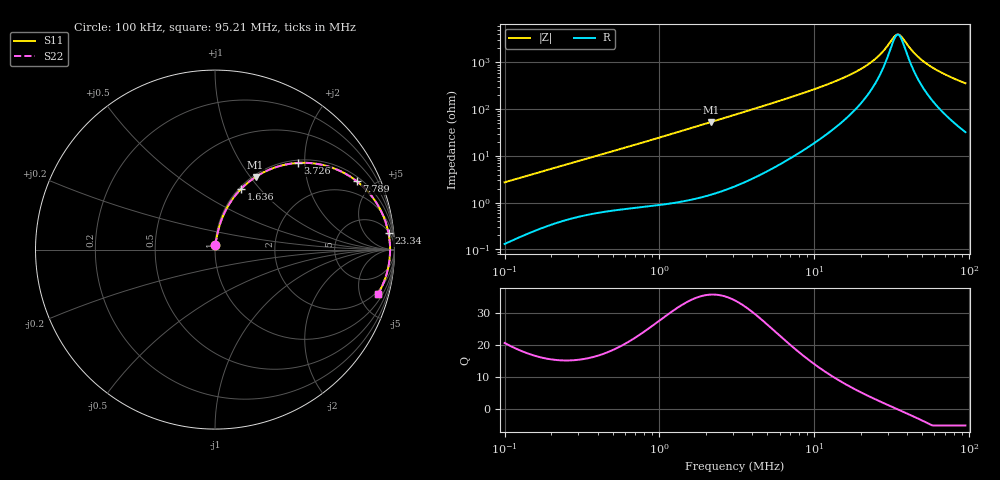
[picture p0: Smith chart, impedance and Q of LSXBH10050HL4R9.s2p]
! LSXBH10050HL4R9  S-PARAMETER MODEL  ( General Type )
! Model Generated by TAIYO YUDEN Corporation (http://www.ty-top.com)
! Version 3.0
! TAIYO YUDEN Control No. 180118NI43SB-FBB
! Copyright(c) 2007 TAIYO YUDEN CO.,LTD. All Rights Reserved.
! Product Description (link to TY-COMPAS)
! https://ds.yuden.co.jp/TYCOMPAS/or/detail?pn=LSXBH10050HL4R9N&u=M
! Products Name : Inductors
! Characteristics :
!  Inductance : 4.9 uH , SRF(min) : 23 MHz , DC Resistance(max) : 0.0195 Ohm
!  Rated Current : Saturation :6600 mA , Temp Rise : 6000 mA (40 degC)
!  Case Size : 10.0 x 9.8 / 0.394 x 0.386 [mm/inch] , Thickness : 5 / 0.197 [mm/inch]
!  (Conditions: Temperature = 25 degC , DC Bias Current/Voltage = 0A / 0V)
! External Node Assignments :
!  1  o---GGG---o  2
! GND o---------o GND
! Frequency Range : 0.1MHz  -  95.211795MHz  [ 402 STEP ]
# MHz S RI R 50
! Freq[MHz].  S11 Real  S11 Imag  S21 Real  S21 Imag  S12 Real  S12 Imag  S22 Real  S22 Imag
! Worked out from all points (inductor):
!   401 points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, 100 kHz to 95.21 MHz, reference 50 ohm
!   read as one part in series: L = 4.29 uH near 103.5 kHz
!   highest Q = 35.9 at 2.153 MHz (marker M1), where L = 3.92 uH
!   self-resonance near 34.84 MHz
!   S11 on the Smith chart (normalised r, x): 100 kHz: 1.00, +0.05; 1.636 MHz: 1.02, +0.81; 3.726 MHz: 1.06, +1.85; 7.789 MHz: 1.22, +4.01; 23.34 MHz: 6, +19; 95.21 MHz: 1.65, -7.16
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0.1  0.00205 0.0271  0.998 -0.0271  0.998 -0.0271  0.00205 0.0271
0.31545  0.0116 0.0796  0.9884 -0.0796  0.9884 -0.0796  0.0116 0.0796
0.574865  0.0269 0.1387  0.9731 -0.1387  0.9731 -0.1387  0.0269 0.1387
0.995088  0.0643 0.2279  0.9357 -0.2279  0.9357 -0.2279  0.0643 0.2279
1.636125  0.1468 0.3396  0.8532 -0.3396  0.8532 -0.3396  0.1468 0.3396
2.152604  0.2258 0.4044  0.7742 -0.4044  0.7742 -0.4044  0.2258 0.4044
3.085641  0.3713 0.4687  0.6287 -0.4687  0.6287 -0.4687  0.3713 0.4687
3.726142  0.4617 0.4829  0.5383 -0.4829  0.5383 -0.4829  0.4617 0.4829
5.250418  0.6291 0.4639  0.3709 -0.4639  0.3709 -0.4639  0.6291 0.4639
7.788765  0.7885 0.382  0.2115 -0.382  0.2115 -0.382  0.7885 0.382
9.733658  0.8533 0.3213  0.1467 -0.3213  0.1467 -0.3213  0.8533 0.3213
16.28088  0.9408 0.1797  0.0592 -0.1797  0.0592 -0.1797  0.9408 0.1797
23.33776  0.9668 0.0909  0.0332 -0.0909  0.0332 -0.0909  0.9668 0.0909
27.23201  0.9723 0.0553  0.0277 -0.0553  0.0277 -0.0553  0.9723 0.0553
30.70484  0.9746 0.0282  0.0254 -0.0282  0.0254 -0.0282  0.9746 0.0282
33.45341  0.9754 0.00906  0.0246 -0.00906  0.0246 -0.00906  0.9754 0.00906
34.62054  0.9755 0.00142  0.0245 -0.00142  0.0245 -0.00142  0.9755 0.00142
35.82839  0.9755 -0.00623  0.0245 0.00623  0.0245 0.00623  0.9755 -0.00623
44.77492  0.9723 -0.0563  0.0277 0.0563  0.0277 0.0563  0.9723 -0.0563
53.14985  0.966 -0.096  0.034 0.096  0.034 0.096  0.966 -0.096
68.73896  0.9489 -0.159  0.0511 0.159  0.0511 0.159  0.9489 -0.159
95.21179  0.9091 -0.2458  0.0909 0.2458  0.0909 0.2458  0.9091 -0.2458
